| IBIS file stm32h562_563_573_lqfp176.ibs
[IBIS ver] 4.2
[File name] stm32h562_563_573_lqfp176.ibs
[File Rev] 1.1
[Date] 07-05-2024
[Source] Data Created at STMicroelectronics
[Notes]  File originated from ELDO simulations.
[Disclaimer]  This information is for modeling purpose only and is
   not guaranteed. The information is subject to change without
   notice.
[Copyright] Copyright 2024 STMicroelectronics Inc.
|   Component stm32h562_563_573_lqfp176
[Component] stm32h562_563_573_lqfp176
[Manufacturer] STMicroelectronics
[Package]
| variable   typ   min   max
R_pkg  0  NA  NA
L_pkg  0  NA  NA
C_pkg  0  NA  NA
[Pin]   signal_name   model_name
1  PE2  io8_ft_i3c_spi
2  PE3  io8_ft_i3c_spi
3  PE4  io8_ft_i3c_spi
4  PE5  io8_ft_i3c_spi
5  PE6  io8_ft_i3c_spi
6  VBAT  power
7  PI8  io8_ft_i3c_spi
8  PC13  io8_ft_i3c_spi
9  PC14-OSC32_IN  io8_ft_i3c_spi
10  PC15-OSC32_OUT  io8_ft_i3c_spi
11  PI9  io8_ft_i3c_spi
12  PI10  io8_ft_i3c_spi
13  PI11  io8_ft_i3c_spi
14  VSS  gnd
15  VDD  power
16  PF0  io8_ft_i3c_spi
17  PF1  io8_ft_i3c_spi
18  PF2  io8_ft_i3c_spi
19  PF3  io8_ft_i3c_spi
20  PF4  io8_ft_i3c_spi
21  PF5  io8_ft_i3c_spi
22  VSS  gnd
23  VDD  power
24  PF6  io8_ft_i3c_spi
25  PF7  io8_ft_i3c_spi
26  PF8  io8_ft_i3c_spi
27  PF9  io8_ft_i3c_spi
28  PF10  io8_ft_i3c_spi
29  PH0-OSC_IN  io8_ft_i3c_spi
30  PH1-OSC_OUT  io8_ft_i3c_spi
31  NRST  ioreset_ft_v33
32  PC0  io8_ft_spi
33  PC1  io8_ft_spi
34  PC2  io8_ft_spi
35  PC3  io8_ft_spi
36  VDD  power
37  VSSA  nc
38  VREFP  nc
39  VDDA  nc
40  PA0  io8_ft_spi
41  PA1  io8_ft_spi_tamp
42  PA2  io8_ft_spi
43  PH2  io8_ft_i3c_spi
44  PH3  io8_ft_i3c_spi
45  PH4  io8_ft_i3c_spi
46  PH5  io8_ft_i3c_spi
47  PA3  io8_ft_spi
48  VSS  gnd
49  VDD  power
50  PA4  io8_ft_spi
51  PA5  io8_ft_spi
52  PA6  io8_ft_spi
53  PA7  io8_ft_spi
54  PC4  io8_ft_spi
55  PC5  io8_ft_spi
56  PB0  io8_ft_spi
57  PB1  io8_ft_spi
58  PB2  io8_ft_i3c_spi
59  PF11  io8_ft_spi
60  PF12  io8_ft_spi
61  VSS  gnd
62  VDD  power
63  PF13  io8_ft_spi
64  PF14  io8_ft_spi
65  PF15  io8_ft_i3c_spi
66  PG0  io8_ft_i3c_spi
67  PG1  io8_ft_i3c_spi
68  PE7  io8_ft_i3c_spi
69  PE8  io8_ft_i3c_spi
70  PE9  io8_ft_i3c_spi
71  VSS  gnd
72  VDD  power
73  PE10  io8_ft_i3c_spi
74  PE11  io8_ft_i3c_spi
75  PE12  io8_ft_i3c_spi
76  PE13  io8_ft_i3c_spi
77  PE14  io8_ft_i3c_spi
78  PE15  io8_ft_i3c_spi
79  PB10  io8_ft_i3c_spi
80  PB11  io8_ft_i3c_spi
81  VCAP  nc
82  VSS  gnd
83  VDD  power
84  PH6  io8_ft_i3c_spi
85  PH7  io8_ft_i3c_spi
86  PH8  io8_ft_i3c_spi
87  PH9  io8_ft_i3c_spi
88  PH10  io8_ft_i3c_spi
89  PH11  io8_ft_i3c_spi
90  PH12  io8_ft_i3c_spi
91  VDD  power
92  PB12  io8_ft_i3c_spi
|93  PB13  io8usb_ft_pd
|94  PB14  io8usb_ft_pd
93 PB13 nc
94 PB14 nc
95  PB15  io8_ft_spi
96  PD8  io8_ft_i3c_spi
97  PD9  io8_ft_i3c_spi
98  PD10  io8_ft_i3c_spi
99  PD11  io8_ft_i3c_spi
100  PD12  io8_ft_i3c_spi
101  PD13  io8_ft_i3c_spi
102  VSS  gnd
103  VDD  power
104  PD14  io8_ft_i3c_spi
105  PD15  io8_ft_i3c_spi
106  PG2  io8_ft_i3c_spi
107  PG3  io8_ft_i3c_spi
108  PG4  io8_ft_i3c_spi
109  PG5  io8_ft_i3c_spi
110  PG6  io8_ft_i3c_spi
111  PG7  io8_ft_i3c_spi
112  PG8  io8_ft_i3c_spi
113  VSS  gnd
114  VDD  power
115  PC6  io8_ft_i3c_spi
116  PC7  io8_ft_i3c_spi
117  PC8  io8_ft_i3c_spi
118  PC9  io8_ft_i3c_spi
119  PA8  io8_ft_i3c_spi
120  PA9  io8_ft_i3c_spi
121  PA10  io8_ft_i3c_spi
122  PA11  io8usb_ft_i3c_spi_phy
123  PA12  io8usb_ft_i3c_spi_phy
124  PA13  io8_ft_i3c_spi
125  VDDUSB  power
126  VSS  gnd
127  VDD  power
128  PH13  io8_ft_i3c_spi
129  PH14  io8_ft_i3c_spi
130  PH15  io8_ft_i3c_spi
131  PI0  io8_ft_i3c_spi
132  PI1  io8_ft_i3c_spi
133  PI2  io8_ft_i3c_spi
134  PI3  io8_ft_i3c_spi
135  VSS  gnd
136  VDD  power
137  PA14  io8_ft_i3c_spi
138  PA15  io8_ft_i3c_spi
139  PC10  io8_ft_i3c_spi
140  PC11  io8_ft_i3c_spi
141  PC12  io8_ft_i3c_spi
142  PD0  io8_ft_i3c_spi
143  PD1  io8_ft_i3c_spi
144  PD2  io8_ft_i3c_spi
145  PD3  io8_ft_i3c_spi
146  PD4  io8_ft_i3c_spi
147  PD5  io8_ft_i3c_spi
148  VSS  gnd
149  VDDIO2  power
150  PD6  io8_ft_i3c_spi
151  PD7  io8_ft_i3c_spi
152  PG9  io8_ft_i3c_spi
153  PG10  io8_ft_i3c_spi
154  PG11  io8_ft_i3c_spi
155  PG12  io8_ft_i3c_spi
156  PG13  io8_ft_i3c_spi
157  PG14  io8_ft_i3c_spi
158  VSS  gnd
159  VDD  power
160  PG15  io8_ft_i3c_spi
161  PB3  io8_ft_i3c_spi
162  PB4  io8_ft_i3c_spi
163  PB5  io8_ft_i3c_spi
164  PB6  io8_ft_i3c_spi
165  PB7  io8_ft_i3c_spi
166  BOOT0  vpphv
167  PB8  io8_ft_i3c_spi
168  PB9  io8_ft_i3c_spi
169  PE0  io8_ft_i3c_spi
170  PE1  io8_ft_i3c_spi
171  VCAP  nc
172  VDD  power
173  PI4  io8_ft_i3c_spi
174  PI5  io8_ft_i3c_spi
175  PI6  io8_ft_i3c_spi
176  PI7  io8_ft_i3c_spi
[Package Model]   484-lqfp-24x24-176-ldo-221014
[Pin Mapping]   pulldown_ref   pullup_ref   | Comment
1  gndio  vddiom
2  gndio  vddiom
3  gndio  vddiom
4  gndio  vddiom
5  gndio  vddiom
6  nc  vsw
7  gndio  vddiom  | Depending on IO usage
| 7  gndio  vsw  | Depending on IO usage
8  gndio  vddiom  | Depending on IO usage
| 8  gndio  vsw  | Depending on IO usage
9  gndio  vddiom  | Depending on IO usage
| 9  gndio  vsw  | Depending on IO usage
10  gndio  vddiom  | Depending on IO usage
| 10  gndio  vsw  | Depending on IO usage
11  gndio  vddiom
12  gndio  vddiom
13  gndio  vddiom
14  gndio  nc
15  nc  vddiom
16  gndio  vddiom
17  gndio  vddiom
18  gndio  vddiom
19  gndio  vddiom
20  gndio  vddiom
21  gndio  vddiom
22  gndio  nc
23  nc  vddiom
24  gndio  vddiom
25  gndio  vddiom
26  gndio  vddiom
27  gndio  vddiom
28  gndio  vddiom
29  gndio  vddiom
30  gndio  vddiom
31  gndio  vddiom
32  gndio  vddiom
33  gndio  vddiom
34  gndio  vddiom
35  gndio  vddiom
36  nc  vddiom
37  nc  nc
38  nc  nc
39  nc  nc
40  gndio  vddiom
41  gndio  vddiom
42  gndio  vddiom
43  gndio  vddiom
44  gndio  vddiom
45  gndio  vddiom
46  gndio  vddiom
47  gndio  vddiom
48  gndio  nc
49  nc  vddiom
50  gndio  vddiom
51  gndio  vddiom
52  gndio  vddiom
53  gndio  vddiom
54  gndio  vddiom
55  gndio  vddiom
56  gndio  vddiom
57  gndio  vddiom
58  gndio  vddiom
59  gndio  vddiom
60  gndio  vddiom
61  gndio  nc
62  nc  vddiom
63  gndio  vddiom
64  gndio  vddiom
65  gndio  vddiom
66  gndio  vddiom
67  gndio  vddiom
68  gndio  vddiom
69  gndio  vddiom
70  gndio  vddiom
71  gndio  nc
72  nc  vddiom
73  gndio  vddiom
74  gndio  vddiom
75  gndio  vddiom
76  gndio  vddiom
77  gndio  vddiom
78  gndio  vddiom
79  gndio  vddiom
80  gndio  vddiom
81  nc  nc
82  gndio  nc
83  nc  vddiom
84  gndio  vddiom
85  gndio  vddiom
86  gndio  vddiom
87  gndio  vddiom
88  gndio  vddiom
89  gndio  vddiom
90  gndio  vddiom
91  nc  vddiom
92  gndio  vddiom
|93  gndio  vddiom
|94  gndio  vddiom
93 nc nc
94 nc nc
95  gndio  vddiom
96  gndio  vddiom
97  gndio  vddiom
98  gndio  vddiom
99  gndio  vddiom
100  gndio  vddiom
101  gndio  vddiom
102  gndio  nc
103  nc  vddiom
104  gndio  vddiom
105  gndio  vddiom
106  gndio  vddiom
107  gndio  vddiom
108  gndio  vddiom
109  gndio  vddiom
110  gndio  vddiom
111  gndio  vddiom
112  gndio  vddiom
113  gndio  nc
114  nc  vddiom
115  gndio  vddiom
116  gndio  vddiom
117  gndio  vddiom
118  gndio  vddiom
119  gndio  vddiom
120  gndio  vddiom  | Depending on IO usage
| 120  gndio  vddusb  | Depending on IO usage
121  gndio  vddiom  | Depending on IO usage
| 121  gndio  vddusb  | Depending on IO usage
122  gndio  vddiom  | Depending on IO usage
| 122  gndio  vddusb  | Depending on IO usage
123  gndio  vddiom  | Depending on IO usage
| 123  gndio  vddusb  | Depending on IO usage
124  gndio  vddiom  | Depending on IO usage
| 124  gndio  vddusb  | Depending on IO usage
125  nc  vddusb
126  gndio  nc
127  nc  vddiom
128  gndio  vddiom
129  gndio  vddiom
130  gndio  vddiom
131  gndio  vddiom
132  gndio  vddiom
133  gndio  vddiom
134  gndio  vddiom
135  gndio  nc
136  nc  vddiom
137  gndio  vddiom
138  gndio  vddiom
139  gndio  vddiom
140  gndio  vddiom
141  gndio  vddiom
142  gndio  vddiom
143  gndio  vddiom
144  gndio  vddiom
145  gndio  vddiom
146  gndio  vddiom
147  gndio  vddiom
148  gndio  nc
149  nc  vddmmc
150  gndio  vddiom  | Depending on IO usage
| 150  gndio  vddmmc  | Depending on IO usage
151  gndio  vddiom  | Depending on IO usage
| 151  gndio  vddmmc  | Depending on IO usage
152  gndio  vddiom  | Depending on IO usage
| 152  gndio  vddmmc  | Depending on IO usage
153  gndio  vddiom  | Depending on IO usage
| 153  gndio  vddmmc  | Depending on IO usage
154  gndio  vddiom  | Depending on IO usage
| 154  gndio  vddmmc  | Depending on IO usage
155  gndio  vddiom  | Depending on IO usage
| 155  gndio  vddmmc  | Depending on IO usage
156  gndio  vddiom  | Depending on IO usage
| 156  gndio  vddmmc  | Depending on IO usage
157  gndio  vddiom  | Depending on IO usage
| 157  gndio  vddmmc  | Depending on IO usage
158  gndio  nc
159  nc  vddiom
160  gndio  vddiom  | Depending on IO usage
| 160  gndio  vddmmc  | Depending on IO usage
161  gndio  vddiom  | Depending on IO usage
| 161  gndio  vddmmc  | Depending on IO usage
162  gndio  vddiom  | Depending on IO usage
| 162  gndio  vddmmc  | Depending on IO usage
163  gndio  vddiom  | Depending on IO usage
| 163  gndio  vddmmc  | Depending on IO usage
164  gndio  vddiom  | Depending on IO usage
| 164  gndio  vddmmc  | Depending on IO usage
165  gndio  vddiom  | Depending on IO usage
| 165  gndio  vddmmc  | Depending on IO usage
166  gndio  vddiom  | Depending on IO usage
| 166  gndio  vddmmc  | Depending on IO usage
167  gndio  vddiom  | Depending on IO usage
| 167  gndio  vddmmc  | Depending on IO usage
168  gndio  vddiom  | Depending on IO usage
| 168  gndio  vddmmc  | Depending on IO usage
169  gndio  vddiom  | Depending on IO usage
| 169  gndio  vddmmc  | Depending on IO usage
170  gndio  vddiom  | Depending on IO usage
| 170  gndio  vddmmc  | Depending on IO usage
171  nc  nc
172  nc  vddiom
173  gndio  vddiom
174  gndio  vddiom
175  gndio  vddiom
176  gndio  vddiom
[Model Selector] io8_ft_i3c_spi
io8_ft_spi_ls_1v2 "io8_ft spi low speed @ 1.2V"
io8_ft_spi_ls_1v8 "io8_ft spi low speed @ 1.8V"
io8_ft_spi_ls_3v3 "io8_ft spi low speed @ 3.3V"
io8_ft_spi_ms_1v2 "io8_ft spi med speed @ 1.2V"
io8_ft_spi_ms_1v8 "io8_ft spi med speed @ 1.8V"
io8_ft_spi_ms_3v3 "io8_ft spi med speed @ 3.3V"
io8_ft_spi_fs_1v2 "io8_ft spi fast speed @ 1.2V"
io8_ft_spi_fs_1v8 "io8_ft spi fast speed @ 1.8V"
io8_ft_spi_fs_3v3 "io8_ft spi fast speed @ 3.3V"
io8_ft_spi_hs_1v2 "io8_ft spi high speed @ 1.2V"
io8_ft_spi_hs_1v8 "io8_ft spi high speed @ 1.8V"
io8_ft_spi_hs_3v3 "io8_ft spi high speed @ 3.3V"
io8_ft_hslv_spi_ls_1v2 "io8_ft spi hslv low speed @ 1.2V"
io8_ft_hslv_spi_ls_1v8 "io8_ft spi hslv low speed @ 1.8V"
io8_ft_hslv_spi_ls_2v5 "io8_ft spi hslv low speed @ 2.5V"
io8_ft_hslv_spi_ms_1v2 "io8_ft spi hslv med speed @ 1.2V"
io8_ft_hslv_spi_ms_1v8 "io8_ft spi hslv med speed @ 1.8V"
io8_ft_hslv_spi_ms_2v5 "io8_ft spi hslv med speed @ 2.5V"
io8_ft_hslv_spi_fs_1v2 "io8_ft spi hslv fast speed @ 1.2V"
io8_ft_hslv_spi_fs_1v8 "io8_ft spi hslv fast speed @ 1.8V"
io8_ft_hslv_spi_fs_2v5 "io8_ft spi hslv fast speed @ 2.5V"
io8_ft_hslv_spi_hs_1v2 "io8_ft spi hslv high speed @ 1.2V"
io8_ft_hslv_spi_hs_1v8 "io8_ft spi hslv high speed @ 1.8V"
io8_ft_hslv_spi_hs_2v5 "io8_ft spi hslv high speed @ 2.5V"
io8_ft_i3c_spi_ls_1v2 "io8_ft i3c spi open-drain low speed @ 1.2V"
io8_ft_i3c_spi_ls_1v8 "io8_ft i3c spi open-drain low speed @ 1.8V"
io8_ft_i3c_spi_ls_3v3 "io8_ft i3c spi open-drain low speed @ 3.3V"
io8_ft_i3c_spi_ms_1v2 "io8_ft i3c spi open-drain med speed @ 1.2V"
io8_ft_i3c_spi_ms_1v8 "io8_ft i3c spi open-drain med speed @ 1.8V"
io8_ft_i3c_spi_ms_3v3 "io8_ft i3c spi open-drain med speed @ 3.3V"
io8_ft_i3c_spi_fs_1v2 "io8_ft i3c spi open-drain fast speed @ 1.2V"
io8_ft_i3c_spi_fs_1v8 "io8_ft i3c spi open-drain fast speed @ 1.8V"
io8_ft_i3c_spi_fs_3v3 "io8_ft i3c spi open-drain fast speed @ 3.3V"
io8_ft_i3c_spi_hs_1v2 "io8_ft i3c spi open-drain high speed @ 1.2V"
io8_ft_i3c_spi_hs_1v8 "io8_ft i3c spi open-drain high speed @ 1.8V"
io8_ft_i3c_spi_hs_3v3 "io8_ft i3c spi open-drain high speed @ 3.3V"
io8_ft_hslv_i3c_spi_ls_1v2 "io8_ft hslv i3c spi open-drain low speed @ 1.2V"
io8_ft_hslv_i3c_spi_ls_1v8 "io8_ft hslv i3c spi open-drain low speed @ 1.8V"
io8_ft_hslv_i3c_spi_ls_2v5 "io8_ft hslv i3c spi open-drain low speed @ 2.5V"
io8_ft_hslv_i3c_spi_ms_1v2 "io8_ft hslv i3c spi open-drain med speed @ 1.2V"
io8_ft_hslv_i3c_spi_ms_1v8 "io8_ft hslv i3c spi open-drain med speed @ 1.8V"
io8_ft_hslv_i3c_spi_ms_2v5 "io8_ft hslv i3c spi open-drain med speed @ 2.5V"
io8_ft_hslv_i3c_spi_fs_1v2 "io8_ft hslv i3c spi open-drain fast speed @ 1.2V"
io8_ft_hslv_i3c_spi_fs_1v8 "io8_ft hslv i3c spi open-drain fast speed @ 1.8V"
io8_ft_hslv_i3c_spi_fs_2v5 "io8_ft hslv i3c spi open-drain fast speed @ 2.5V"
io8_ft_hslv_i3c_spi_hs_1v2 "io8_ft hslv i3c spi open-drain high speed @ 1.2V"
io8_ft_hslv_i3c_spi_hs_1v8 "io8_ft hslv i3c spi open-drain high speed @ 1.8V"
io8_ft_hslv_i3c_spi_hs_2v5 "io8_ft hslv i3c spi open-drain high speed @ 2.5V"
io8_ft_i3c_fmp_spi_3v3 "io8_ft i3c fm+ spi open-drain @ 3.3V"
io8_ft_i3c_fmp_spi_1v8 "io8_ft i3c fm+ spi open-drain @ 1.8V"
io8_ft_i3c_fmp_spi_1v2 "io8_ft i3c fm+ spi open-drain @ 1.2V"
[Model Selector] io8_ft_spi
io8_ft_spi_ls_1v2 "io8_ft spi low speed @ 1.2V"
io8_ft_spi_ls_1v8 "io8_ft spi low speed @ 1.8V"
io8_ft_spi_ls_3v3 "io8_ft spi low speed @ 3.3V"
io8_ft_spi_ms_1v2 "io8_ft spi med speed @ 1.2V"
io8_ft_spi_ms_1v8 "io8_ft spi med speed @ 1.8V"
io8_ft_spi_ms_3v3 "io8_ft spi med speed @ 3.3V"
io8_ft_spi_fs_1v2 "io8_ft spi fast speed @ 1.2V"
io8_ft_spi_fs_1v8 "io8_ft spi fast speed @ 1.8V"
io8_ft_spi_fs_3v3 "io8_ft spi fast speed @ 3.3V"
io8_ft_spi_hs_1v2 "io8_ft spi high speed @ 1.2V"
io8_ft_spi_hs_1v8 "io8_ft spi high speed @ 1.8V"
io8_ft_spi_hs_3v3 "io8_ft spi high speed @ 3.3V"
io8_ft_hslv_spi_ls_1v2 "io8_ft spi hslv low speed @ 1.2V"
io8_ft_hslv_spi_ls_1v8 "io8_ft spi hslv low speed @ 1.8V"
io8_ft_hslv_spi_ls_2v5 "io8_ft spi hslv low speed @ 2.5V"
io8_ft_hslv_spi_ms_1v2 "io8_ft spi hslv med speed @ 1.2V"
io8_ft_hslv_spi_ms_1v8 "io8_ft spi hslv med speed @ 1.8V"
io8_ft_hslv_spi_ms_2v5 "io8_ft spi hslv med speed @ 2.5V"
io8_ft_hslv_spi_fs_1v2 "io8_ft spi hslv fast speed @ 1.2V"
io8_ft_hslv_spi_fs_1v8 "io8_ft spi hslv fast speed @ 1.8V"
io8_ft_hslv_spi_fs_2v5 "io8_ft spi hslv fast speed @ 2.5V"
io8_ft_hslv_spi_hs_1v2 "io8_ft spi hslv high speed @ 1.2V"
io8_ft_hslv_spi_hs_1v8 "io8_ft spi hslv high speed @ 1.8V"
io8_ft_hslv_spi_hs_2v5 "io8_ft spi hslv high speed @ 2.5V"
[Model Selector] io8_ft_spi_tamp
io8_ft_spi_ls_1v2 "io8_ft spi low speed @ 1.2V"
io8_ft_spi_ls_1v8 "io8_ft spi low speed @ 1.8V"
io8_ft_spi_ls_3v3 "io8_ft spi low speed @ 3.3V"
io8_ft_spi_ms_1v2 "io8_ft spi med speed @ 1.2V"
io8_ft_spi_ms_1v8 "io8_ft spi med speed @ 1.8V"
io8_ft_spi_ms_3v3 "io8_ft spi med speed @ 3.3V"
io8_ft_spi_fs_1v2 "io8_ft spi fast speed @ 1.2V"
io8_ft_spi_fs_1v8 "io8_ft spi fast speed @ 1.8V"
io8_ft_spi_fs_3v3 "io8_ft spi fast speed @ 3.3V"
io8_ft_spi_hs_1v2 "io8_ft spi high speed @ 1.2V"
io8_ft_spi_hs_1v8 "io8_ft spi high speed @ 1.8V"
io8_ft_spi_hs_3v3 "io8_ft spi high speed @ 3.3V"
io8_ft_hslv_spi_ls_1v2 "io8_ft spi hslv low speed @ 1.2V"
io8_ft_hslv_spi_ls_1v8 "io8_ft spi hslv low speed @ 1.8V"
io8_ft_hslv_spi_ls_2v5 "io8_ft spi hslv low speed @ 2.5V"
io8_ft_hslv_spi_ms_1v2 "io8_ft spi hslv med speed @ 1.2V"
io8_ft_hslv_spi_ms_1v8 "io8_ft spi hslv med speed @ 1.8V"
io8_ft_hslv_spi_ms_2v5 "io8_ft spi hslv med speed @ 2.5V"
io8_ft_hslv_spi_fs_1v2 "io8_ft spi hslv fast speed @ 1.2V"
io8_ft_hslv_spi_fs_1v8 "io8_ft spi hslv fast speed @ 1.8V"
io8_ft_hslv_spi_fs_2v5 "io8_ft spi hslv fast speed @ 2.5V"
io8_ft_hslv_spi_hs_1v2 "io8_ft spi hslv high speed @ 1.2V"
io8_ft_hslv_spi_hs_1v8 "io8_ft spi hslv high speed @ 1.8V"
io8_ft_hslv_spi_hs_2v5 "io8_ft spi hslv high speed @ 2.5V"
io8_ft_tamp_v33_1v2 "io8_ft tamp V33 @ 1.2V"
io8_ft_tamp_v33_1v8 "io8_ft tamp V33 @ 1.2V"
io8_ft_tamp_v33_3v3 "io8_ft tamp V33 @ 1.2V"
[Model Selector] io8usb_ft_i3c_spi_phy
io8_ft_spi_ls_1v2 "io8_ft spi low speed @ 1.2V"
io8_ft_spi_ls_1v8 "io8_ft spi low speed @ 1.8V"
io8_ft_spi_ls_3v3 "io8_ft spi low speed @ 3.3V"
io8_ft_spi_ms_1v2 "io8_ft spi med speed @ 1.2V"
io8_ft_spi_ms_1v8 "io8_ft spi med speed @ 1.8V"
io8_ft_spi_ms_3v3 "io8_ft spi med speed @ 3.3V"
io8_ft_spi_fs_1v2 "io8_ft spi fast speed @ 1.2V"
io8_ft_spi_fs_1v8 "io8_ft spi fast speed @ 1.8V"
io8_ft_spi_fs_3v3 "io8_ft spi fast speed @ 3.3V"
io8_ft_spi_hs_1v2 "io8_ft spi high speed @ 1.2V"
io8_ft_spi_hs_1v8 "io8_ft spi high speed @ 1.8V"
io8_ft_spi_hs_3v3 "io8_ft spi high speed @ 3.3V"
io8_ft_hslv_spi_ls_1v2 "io8_ft spi hslv low speed @ 1.2V"
io8_ft_hslv_spi_ls_1v8 "io8_ft spi hslv low speed @ 1.8V"
io8_ft_hslv_spi_ls_2v5 "io8_ft spi hslv low speed @ 2.5V"
io8_ft_hslv_spi_ms_1v2 "io8_ft spi hslv med speed @ 1.2V"
io8_ft_hslv_spi_ms_1v8 "io8_ft spi hslv med speed @ 1.8V"
io8_ft_hslv_spi_ms_2v5 "io8_ft spi hslv med speed @ 2.5V"
io8_ft_hslv_spi_fs_1v2 "io8_ft spi hslv fast speed @ 1.2V"
io8_ft_hslv_spi_fs_1v8 "io8_ft spi hslv fast speed @ 1.8V"
io8_ft_hslv_spi_fs_2v5 "io8_ft spi hslv fast speed @ 2.5V"
io8_ft_hslv_spi_hs_1v2 "io8_ft spi hslv high speed @ 1.2V"
io8_ft_hslv_spi_hs_1v8 "io8_ft spi hslv high speed @ 1.8V"
io8_ft_hslv_spi_hs_2v5 "io8_ft spi hslv high speed @ 2.5V"
io8_ft_i3c_spi_ls_1v2 "io8_ft i3c spi open-drain low speed @ 1.2V"
io8_ft_i3c_spi_ls_1v8 "io8_ft i3c spi open-drain low speed @ 1.8V"
io8_ft_i3c_spi_ls_3v3 "io8_ft i3c spi open-drain low speed @ 3.3V"
io8_ft_i3c_spi_ms_1v2 "io8_ft i3c spi open-drain med speed @ 1.2V"
io8_ft_i3c_spi_ms_1v8 "io8_ft i3c spi open-drain med speed @ 1.8V"
io8_ft_i3c_spi_ms_3v3 "io8_ft i3c spi open-drain med speed @ 3.3V"
io8_ft_i3c_spi_fs_1v2 "io8_ft i3c spi open-drain fast speed @ 1.2V"
io8_ft_i3c_spi_fs_1v8 "io8_ft i3c spi open-drain fast speed @ 1.8V"
io8_ft_i3c_spi_fs_3v3 "io8_ft i3c spi open-drain fast speed @ 3.3V"
io8_ft_i3c_spi_hs_1v2 "io8_ft i3c spi open-drain high speed @ 1.2V"
io8_ft_i3c_spi_hs_1v8 "io8_ft i3c spi open-drain high speed @ 1.8V"
io8_ft_i3c_spi_hs_3v3 "io8_ft i3c spi open-drain high speed @ 3.3V"
io8_ft_hslv_i3c_spi_ls_1v2 "io8_ft hslv i3c spi open-drain low speed @ 1.2V"
io8_ft_hslv_i3c_spi_ls_1v8 "io8_ft hslv i3c spi open-drain low speed @ 1.8V"
io8_ft_hslv_i3c_spi_ls_2v5 "io8_ft hslv i3c spi open-drain low speed @ 2.5V"
io8_ft_hslv_i3c_spi_ms_1v2 "io8_ft hslv i3c spi open-drain med speed @ 1.2V"
io8_ft_hslv_i3c_spi_ms_1v8 "io8_ft hslv i3c spi open-drain med speed @ 1.8V"
io8_ft_hslv_i3c_spi_ms_2v5 "io8_ft hslv i3c spi open-drain med speed @ 2.5V"
io8_ft_hslv_i3c_spi_fs_1v2 "io8_ft hslv i3c spi open-drain fast speed @ 1.2V"
io8_ft_hslv_i3c_spi_fs_1v8 "io8_ft hslv i3c spi open-drain fast speed @ 1.8V"
io8_ft_hslv_i3c_spi_fs_2v5 "io8_ft hslv i3c spi open-drain fast speed @ 2.5V"
io8_ft_hslv_i3c_spi_hs_1v2 "io8_ft hslv i3c spi open-drain high speed @ 1.2V"
io8_ft_hslv_i3c_spi_hs_1v8 "io8_ft hslv i3c spi open-drain high speed @ 1.8V"
io8_ft_hslv_i3c_spi_hs_2v5 "io8_ft hslv i3c spi open-drain high speed @ 2.5V"
io8_ft_i3c_fmp_spi_3v3 "io8_ft i3c fm+ spi open-drain @ 3.3V"
io8_ft_i3c_fmp_spi_1v8 "io8_ft i3c fm+ spi open-drain @ 1.8V"
io8_ft_i3c_fmp_spi_1v2 "io8_ft i3c fm+ spi open-drain @ 1.2V"
io8usb_ft_phy_ls_2v5 "iousb ft low speed @ 2.5V"
io8usb_ft_phy_ls_3v3 "iousb ft low speed @ 3.3V"
io8usb_ft_phy_fs_2v5 "iousb ft fast speed @ 2.5V"
io8usb_ft_phy_fs_3v3 "iousb ft fast speed @ 3.3V"
[Model Selector] ioreset_ft_v33
ioreset_ft_v33_1v2 "Reset PAD. 5V tolerant. 1.2V range"
ioreset_ft_v33_1v8 "Reset PAD. 5V tolerant. 1.8V range"
ioreset_ft_v33_3v3 "Reset PAD. 5V tolerant. 3.3V range"
[Model Selector] vpphv
vpphv_1v2 "Flash Test cell v33 = 1.2 V range"
vpphv_1v8 "Flash Test cell v33 = 1.8 V range"
vpphv_3v3 "Flash Test cell v33 = 3.3 V range"
[Define Package Model]  484-lqfp-24x24-176-ldo-221014
[Manufacturer]  Unknown
[OEM]  Unknown
[Description]  None
[Number Of Pins]  172
[Pin Numbers]
| Pin Num   Terminal Name
166 | BOOT0
31 | NRST
40 | PA0
41 | PA1
42 | PA2
47 | PA3
50 | PA4
51 | PA5
52 | PA6
53 | PA7
119 | PA8
120 | PA9
121 | PA10
122 | PA11
123 | PA12
124 | PA13
137 | PA14
138 | PA15
56 | PB0
57 | PB1
58 | PB2
161 | PB3
162 | PB4
163 | PB5
164 | PB6
165 | PB7
167 | PB8
168 | PB9
79 | PB10
80 | PB11
92 | PB12
93 | PB13
94 | PB14
95 | PB15
32 | PC0
33 | PC1
34 | PC2
35 | PC3
54 | PC4
55 | PC5
115 | PC6
116 | PC7
117 | PC8
118 | PC9
139 | PC10
140 | PC11
141 | PC12
8 | PC13
9 | PC14-OSC32_IN
10 | PC15-OSC32_OUT
142 | PD0
143 | PD1
144 | PD2
145 | PD3
146 | PD4
147 | PD5
150 | PD6
151 | PD7
96 | PD8
97 | PD9
98 | PD10
99 | PD11
100 | PD12
101 | PD13
104 | PD14
105 | PD15
169 | PE0
170 | PE1
1 | PE2
2 | PE3
3 | PE4
4 | PE5
5 | PE6
68 | PE7
69 | PE8
70 | PE9
73 | PE10
74 | PE11
75 | PE12
76 | PE13
77 | PE14
78 | PE15
16 | PF0
17 | PF1
18 | PF2
19 | PF3
20 | PF4
21 | PF5
24 | PF6
25 | PF7
26 | PF8
27 | PF9
28 | PF10
59 | PF11
60 | PF12
63 | PF13
64 | PF14
65 | PF15
66 | PG0
67 | PG1
106 | PG2
107 | PG3
108 | PG4
109 | PG5
110 | PG6
111 | PG7
112 | PG8
152 | PG9
153 | PG10
154 | PG11
155 | PG12
156 | PG13
157 | PG14
160 | PG15
29 | PH0-OSC_IN
30 | PH1-OSC_OUT
43 | PH2
44 | PH3
45 | PH4
46 | PH5
84 | PH6
85 | PH7
86 | PH8
87 | PH9
88 | PH10
89 | PH11
90 | PH12
128 | PH13
129 | PH14
130 | PH15
131 | PI0
132 | PI1
133 | PI2
134 | PI3
173 | PI4
174 | PI5
175 | PI6
176 | PI7
7 | PI8
11 | PI9
12 | PI10
13 | PI11
6 | VBAT
81 | VCAP
171 | VCAP
83 | VDD
127 | VDD
15 | VDD
23 | VDD
36 | VDD
49 | VDD
62 | VDD
72 | VDD
172 | VDD
91 | VDD
103 | VDD
136 | VDD
159 | VDD
114 | VDD
149 | VDDIO2
125 | VDDUSB
39 | VDDA
38 | VREFP
82 | VSS
14 | VSS
61 | VSS
102 | VSS
135 | VSS
148 | VSS
113 | VSS
22 | VSS
37 | VSSA
|[Merged Pins]  22
|48  |  VSS
|71  |  VSS
|126  |  VSS
|158  |  VSS
[Model Data]
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[End Model Data]
[End Package Model]
|End [Component]
| Models and submodels in the file (64): io8_ft_hslv_i3c_spi_fs_1v2 (I/O_open_drain), io8_ft_hslv_i3c_spi_fs_1v8 (I/O_open_drain), io8_ft_hslv_i3c_spi_fs_2v5 (I/O_open_drain), io8_ft_hslv_i3c_spi_hs_1v2 (I/O_open_drain), io8_ft_hslv_i3c_spi_hs_1v8 (I/O_open_drain), io8_ft_hslv_i3c_spi_hs_2v5 (I/O_open_drain), io8_ft_hslv_i3c_spi_ls_1v2 (I/O_open_drain), io8_ft_hslv_i3c_spi_ls_1v8 (I/O_open_drain), io8_ft_hslv_i3c_spi_ls_2v5 (I/O_open_drain), io8_ft_hslv_i3c_spi_ms_1v2 (I/O_open_drain), io8_ft_hslv_i3c_spi_ms_1v8 (I/O_open_drain), io8_ft_hslv_i3c_spi_ms_2v5 (I/O_open_drain), io8_ft_hslv_spi_fs_1v2 (I/O), io8_ft_hslv_spi_fs_1v8 (I/O), io8_ft_hslv_spi_fs_2v5 (I/O), io8_ft_hslv_spi_hs_1v2 (I/O), io8_ft_hslv_spi_hs_1v8 (I/O), io8_ft_hslv_spi_hs_2v5 (I/O), io8_ft_hslv_spi_ls_1v2 (I/O), io8_ft_hslv_spi_ls_1v8 (I/O), io8_ft_hslv_spi_ls_2v5 (I/O), io8_ft_hslv_spi_ms_1v2 (I/O), io8_ft_hslv_spi_ms_1v8 (I/O), io8_ft_hslv_spi_ms_2v5 (I/O), io8_ft_i3c_fmp_spi_1v2 (I/O_open_drain), io8_ft_i3c_fmp_spi_1v8 (I/O_open_drain), io8_ft_i3c_fmp_spi_3v3 (I/O_open_drain), io8_ft_i3c_spi_fs_1v2 (I/O_open_drain), io8_ft_i3c_spi_fs_1v8 (I/O_open_drain), io8_ft_i3c_spi_fs_3v3 (I/O_open_drain), io8_ft_i3c_spi_hs_1v2 (I/O_open_drain), io8_ft_i3c_spi_hs_1v8 (I/O_open_drain), io8_ft_i3c_spi_hs_3v3 (I/O_open_drain), io8_ft_i3c_spi_ls_1v2 (I/O_open_drain), io8_ft_i3c_spi_ls_1v8 (I/O_open_drain), io8_ft_i3c_spi_ls_3v3 (I/O_open_drain), io8_ft_i3c_spi_ms_1v2 (I/O_open_drain), io8_ft_i3c_spi_ms_1v8 (I/O_open_drain), io8_ft_i3c_spi_ms_3v3 (I/O_open_drain), io8_ft_spi_fs_1v2 (I/O), io8_ft_spi_fs_1v8 (I/O), io8_ft_spi_fs_3v3 (I/O), io8_ft_spi_hs_1v2 (I/O), io8_ft_spi_hs_1v8 (I/O), io8_ft_spi_hs_3v3 (I/O), io8_ft_spi_ls_1v2 (I/O), io8_ft_spi_ls_1v8 (I/O), io8_ft_spi_ls_3v3 (I/O), io8_ft_spi_ms_1v2 (I/O), io8_ft_spi_ms_1v8 (I/O), io8_ft_spi_ms_3v3 (I/O), io8_ft_tamp_v33_1v2 (I/O), io8_ft_tamp_v33_1v8 (I/O), io8_ft_tamp_v33_3v3 (I/O), io8usb_ft_phy_fs_2v5 (I/O), io8usb_ft_phy_fs_3v3 (I/O), io8usb_ft_phy_ls_2v5 (I/O), io8usb_ft_phy_ls_3v3 (I/O), ioreset_ft_v33_1v2 (I/O_open_drain), ioreset_ft_v33_1v8 (I/O_open_drain), ioreset_ft_v33_3v3 (I/O_open_drain), vpphv_1v2 (Input), vpphv_1v8 (Input), vpphv_3v3 (Input)
